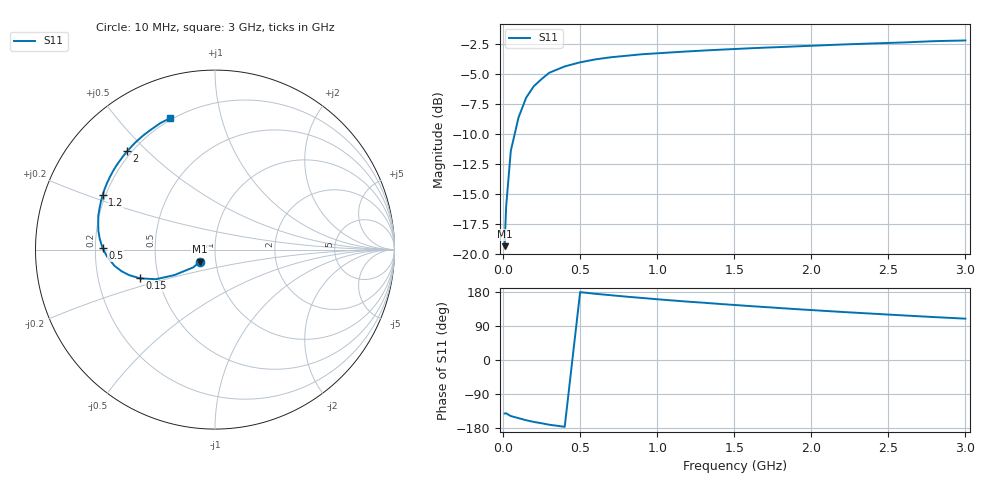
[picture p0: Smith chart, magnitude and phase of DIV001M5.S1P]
! SIEMENS Small Signal Semiconductors
! BAV99
! Silicon Switching Diode in SOT23
! IF = 1.5 mA
! S-Parameters:  May  1995
# GHz  S  MA  R  50
!  f  S11
! GHz  MAG  ANG
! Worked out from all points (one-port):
!   30 points, 10 MHz to 3 GHz, reference 50 ohm
!   lowest |S11| = -19.4 dB at 10 MHz (marker M1), VSWR 1.24, Z = 41.9 - j5.71 ohm
!   |S11| at or under -10 dB: start of sweep to 76.08 MHz
!   S11 on the Smith chart (normalised r, x): 10 MHz: 0.84, -0.11; 150 MHz: 0.39, -0.16; 500 MHz: 0.23, +0.01; 1.2 GHz: 0.19, +0.22; 2 GHz: 0.18, +0.43; 3 GHz: 0.19, +0.69
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0.01  0.1074 -141.2
0.02  0.1573 -140.8
0.05  0.2676 -147.9
0.1  0.3686 -153.4
0.15  0.4467 -159.0
0.2  0.4987 -163.4
0.25  0.5337 -166.9
0.3  0.5671 -170.8
0.4  0.6026 -176.3
0.5  0.6267 179.1
0.6  0.6448 174.7
0.7  0.6581 170.9
0.8  0.6673 167.2
0.9  0.6771 163.8
1  0.6833 160.3
1.1  0.6898 157.1
1.2  0.6959 154.0
1.3  0.7017 151.2
1.4  0.707 148.1
1.6  0.717 142.4
1.7  0.7217 139.7
1.9  0.7302 134.3
2  0.7346 131.8
2.2  0.7436 126.8
2.4  0.7513 122.2
2.6  0.7584 117.6
2.8  0.768 113.2
3  0.773 109.1
